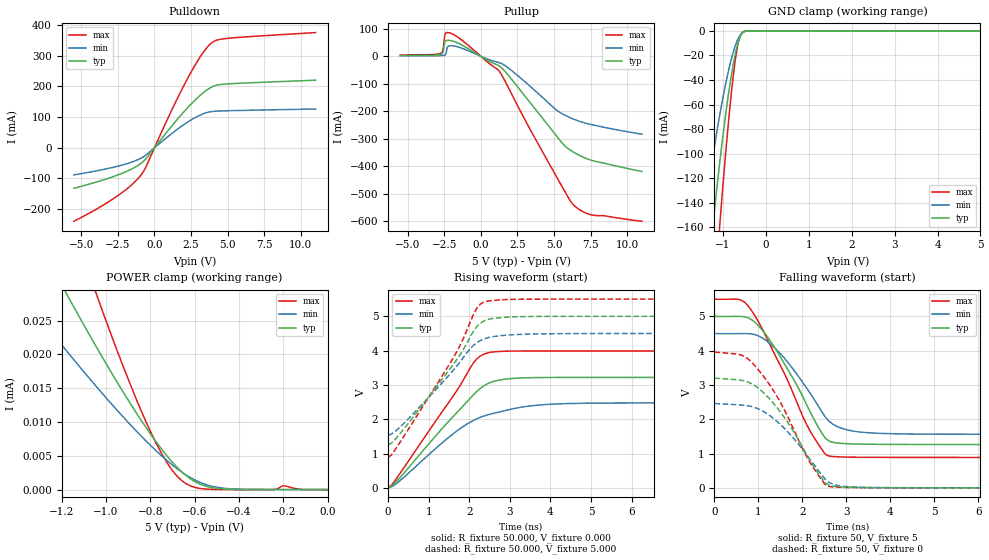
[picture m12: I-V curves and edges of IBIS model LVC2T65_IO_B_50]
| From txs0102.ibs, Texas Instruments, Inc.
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[Model]   LVC2T65_IO_B_50
Model_type  I/O
Vinl=0.15
Vinh=5.1
Enable   Active-High
Vref =   5
Rref =   1000000
Cref =   15p
Vmeas =   2.5
| variable   typ   min   max
C_comp   6.72pF   5.75pF   7.72pF
| C_pullup   6.74pF   5.73pF   7.54pF
| C_pulldown   7.06pF   6.37pF   7.63pF
| C_tri-state   6.72pF   5.75pF   7.72pF
[Temperature Range]   40   100   -40
| Ambient temperature   25   85   -40
[Voltage range]   5   4.5   5.5
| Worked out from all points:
|   slope of the pulldown table from 0 to 0.75 V, typ, clamps not added: 16.4 ohm
|   slope of the pullup table from 0 to 0.75 V, typ, clamps not added: 33.6 ohm
|   GND clamp passes 1 mA (typ) near -0.52 V on its own axis
|   rising waveform, R_fixture 50.000, V_fixture 0.000: 20-80 % time 1.44ns typ, 1.54ns min, 1.36ns max; typ from 0.006 V to 3.2 V
|   falling waveform, R_fixture 50, V_fixture 5: 20-80 % time 975ps typ, 984ps min, 1ns max; typ from 5 V to 1.26 V
|   rising waveform, R_fixture 50.000, V_fixture 5.000: 20-80 % time 1.38ns typ, 1.33ns min, 1.38ns max; typ from 1.25 V to 5 V
|   falling waveform, R_fixture 50, V_fixture 0: 20-80 % time 970ps typ, 975ps min, 985ps max; typ from 3.2 V to 0.006 V
[GND Clamp]
| LVC2T65_IO_B_50
|   Voltage   I(typ)   I(min)   I(max)
-5.5V     -2.167A    -1.64A     -2.768A
-1.46V    -238.9mA   -156.6mA   -348.3mA
-1.235V   -157.8mA   -101.9mA   -233mA
-1.085V   -109.4mA   -69.97mA   -162mA
-1.065V   -103.4mA   -66.03mA   -152.9mA
-900mV    -57.98mA   -36.69mA   -84.14mA
-815mV    -38.17mA   -24.08mA   -53.51mA
-740mV    -23.28mA   -14.75mA   -30.35mA
-685mV    -14.32mA   -9.24mA    -16.88mA
-630mV    -7.509mA   -5.07mA    -7.45mA
-520mV    -1.048mA   -871.9uA   -563uA
5V        652.3pA    345.2nA    120.4pA
[POWER Clamp]
| LVC2T65_IO_B_50
|   Voltage   I(typ)   I(min)   I(max)
-5.5V     342.7uA    230.7uA    551.8uA
-1.395V   42.24uA    29.44uA    63.26uA
-1.35V    39.43uA    27.55uA    58.68uA
-1.2V     30.26uA    21.4uA     43.77uA
-1.15V    27.28uA    19.4uA     38.93uA
-1.05V    21.47uA    15.49uA    29.52uA
-795mV    8.022uA    6.402uA    8.279uA
-725mV    4.985uA    4.3uA      3.995uA
-660mV    2.681uA    2.631uA    1.385uA
-585mV    939.3nA    1.198uA    222.6nA
-500mV    177.3nA    345.2nA    16.11nA
0V        0A         0A         0A
[Pulldown]
| LVC2T65_IO_B_50
|   Voltage   I(typ)   I(min)   I(max)
-5.5V     -131.8mA   -88.38mA   -239.5mA
-2.58V    -90.08mA   -60.91mA   -158.9mA
-1.6V     -70.37mA   -47.47mA   -122.9mA
-925mV    -51.22mA   -34.19mA   -89.37mA
-585mV    -36.39mA   -24.06mA   -63.21mA
1.05V     63.01mA    41.18mA    109.2mA
2.245V    129.3mA    82.9mA     223.9mA
3.2V      173.9mA    108.2mA    301.4mA
3.905V    197.8mA    117.9mA    341.8mA
4.31V     204.6mA    119.5mA    351.3mA
5.045V    208.3mA    120.7mA    356.8mA
11V       220.2mA    126.3mA    375.4mA
[Pullup]
| LVC2T65_IO_B_50
|   Voltage   I(typ)   I(min)   I(max)
-5.5V     3.181mA    1.83mA     4.924mA
-2.795V   6.211mA    2.516mA    9.717mA
-2.595V   13.71mA    3.139mA    21.91mA
-2.46V    51.74mA    4.292mA    76.09mA
-2.4V     55.9mA     6.57mA     84.26mA
-2.22V    58.31mA    36.26mA    86.31mA
-1.55V    47.9mA     34.16mA    69.1mA
1.295V    -36.16mA   -23.98mA   -56.86mA
5.565V    -316.7mA   -209.7mA   -476.1mA
6.34V     -349.4mA   -229.1mA   -541.7mA
7.505V    -377.9mA   -248.1mA   -577mA
11V       -419.5mA   -283.6mA   -601mA
[Ramp]
| LVC2T65_IO_B_50
| variable   typ   min   max
dV/dt_r   2.03/1.45E-09   1.58/1.56E-09   2.50/1.37E-09
dV/dt_f   2.24/9.75E-10   1.77/9.84E-10   2.77/1.00E-09
R_load = 50
[Rising Waveform]
R_fixture = 50.000
V_fixture = 0.000
V_fixture_min = 0.000
V_fixture_max = 0.000
C_fixture = 0.000
L_fixture = 0.000
|  time   V(typ)   V(min)   V(max)
0s        6.037mV    5.33mV     6.518mV
84ps      52.95mV    33.92mV    84.37mV
252ps     249.2mV    173.1mV    353.9mV
1.596ns   2.073V     1.573V     2.666V
2.184ns   2.811V     2.016V     3.76V
2.52ns    3.075V     2.153V     3.954V
3.192ns   3.2V       2.335V     3.989V
4.284ns   3.22V      2.454V     3.99V
6.636ns   3.22V      2.478V     3.989V
419.9ns   3.2V       2.462V     3.957V
[Falling Waveform]
| LVC2T65_IO_B_50
R_fixture =   50
C_fixture =   0
L_fixture =   0
V_fixture =   5
V_fixture_min = 4.5
V_fixture_max = 5.5
|   Time   V(typ)   V(min)   V(max)
0s        5V         4.5V       5.5V
588ps     4.997V     4.495V     5.48V
840ps     4.905V     4.488V     5.175V
1.176ns   4.451V     4.295V     4.401V
1.512ns   3.786V     3.893V     3.533V
2.1ns     2.416V     2.902V     1.837V
2.52ns    1.452V     2.066V     983.2mV
2.772ns   1.314V     1.802V     910.7mV
3.276ns   1.28V      1.635V     895.6mV
419.9ns   1.26V      1.546V     888.3mV
[Rising Waveform]
R_fixture = 50.000
V_fixture = 5.000
V_fixture_min = 4.500
V_fixture_max = 5.500
C_fixture = 0.000
L_fixture = 0.000
|  time   V(typ)   V(min)   V(max)
0s        1.255V     1.54V      884.7mV
84ps      1.306V     1.572V     968.2mV
336ps     1.644V     1.824V     1.409V
1.596ns   3.584V     3.416V     3.77V
1.848ns   4.02V      3.79V      4.34V
2.1ns     4.562V     4.151V     5.048V
2.268ns   4.795V     4.29V      5.35V
2.52ns    4.926V     4.396V     5.452V
3.36ns    4.991V     4.478V     5.498V
419.9ns   5V         4.5V       5.5V
[Falling Waveform]
| LVC2T65_IO_B_50
R_fixture =   50
C_fixture =   0
L_fixture =   0
V_fixture =   0
V_fixture_min = 0
V_fixture_max = 0
|   Time   V(typ)   V(min)   V(max)
0s        3.198V     2.46V      3.957V
672ps     3.123V     2.408V     3.837V
1.008ns   2.894V     2.298V     3.427V
1.344ns   2.463V     2.024V     2.829V
1.68ns    1.884V     1.616V     2.041V
2.1ns     965.1mV    960.5mV    905mV
2.52ns    149.9mV    251.2mV    95.47mV
2.772ns   43.01mV    80.75mV    26.39mV
3.36ns    14.32mV    21.37mV    10.44mV
419.9ns   5.759mV    4.784mV    6.496mV
